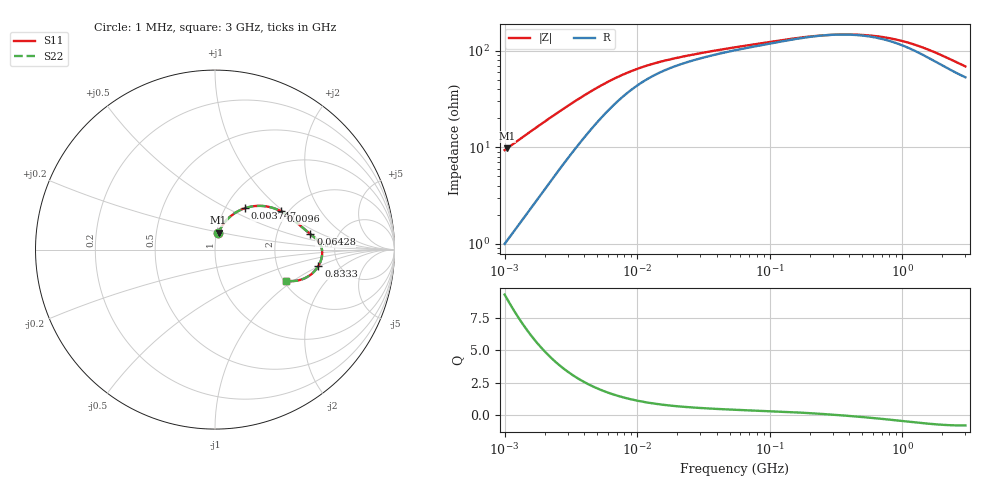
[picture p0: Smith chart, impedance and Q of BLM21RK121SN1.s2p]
! BLM21RK121SN1
# Hz S RI R 50
!Freq.(Hz) S11(Real) S11(Imag) S21(Real) S21(Imag) S12(Real) S12(Imag) S22(Real) S22(Imag)
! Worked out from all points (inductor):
!   401 points, 1 MHz to 3 GHz, reference 50 ohm
!   read as one part in series: L = 1.48 uH near 1.041 MHz
!   highest Q = 9.02 at 1.041 MHz (marker M1), where L = 1.49 uH
!   self-resonance near 308.7 MHz
!   S11 on the Smith chart (normalised r, x): 1 MHz: 1.02, +0.19; 3.747 MHz: 1.23, +0.62; 9.6 MHz: 1.84, +0.96; 64.28 MHz: 3.12, +0.77; 833.3 MHz: 3.50, -0.98; 3 GHz: 2.07, -0.88
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1000000  0.0183 0.0908  0.9817 -0.0908  0.9817 -0.0908  0.0183 0.0908
1040844  0.0197 0.0942  0.9803 -0.0942  0.9803 -0.0942  0.0197 0.0942
1492300  0.0382 0.1296  0.9618 -0.1296  0.9618 -0.1296  0.0382 0.1296
2055611  0.067 0.1668  0.933 -0.1668  0.933 -0.1668  0.067 0.1668
2775447  0.1088 0.2022  0.8912 -0.2022  0.8912 -0.2022  0.1088 0.2022
3747356  0.1662 0.2306  0.8338 -0.2306  0.8338 -0.2306  0.1662 0.2306
3823119  0.1705 0.232  0.8295 -0.232  0.8295 -0.232  0.1705 0.232
4764734  0.2202 0.2425  0.7798 -0.2425  0.7798 -0.2425  0.2202 0.2425
5938264  0.2714 0.2426  0.7286 -0.2426  0.7286 -0.2426  0.2714 0.2426
9600343  0.3682 0.2133  0.6318 -0.2133  0.6318 -0.2133  0.3682 0.2133
1.461624e7  0.4255 0.1754  0.5745 -0.1754  0.5745 -0.1754  0.4255 0.1754
2.509235e7  0.4732 0.1349  0.5268 -0.1349  0.5268 -0.1349  0.4732 0.1349
5.477226e7  0.5225 0.0942  0.4775 -0.0942  0.4775 -0.0942  0.5225 0.0942
6.428402e7  0.5312 0.0872  0.4688 -0.0872  0.4688 -0.0872  0.5312 0.0872
2.094008e8  0.5869 0.0284  0.4131 -0.0284  0.4131 -0.0284  0.5869 0.0284
4.304467e8  0.5968 -0.0277  0.4032 0.0277  0.4032 0.0277  0.5968 -0.0277
8.005644e8  0.5781 -0.088  0.4219 0.088  0.4219 0.088  0.5781 -0.088
8.332625e8  0.5757 -0.0922  0.4243 0.0922  0.4243 0.0922  0.5757 -0.0922
1.218836e9  0.5424 -0.1321  0.4576 0.1321  0.4576 0.1321  0.5424 -0.1321
1.782824e9  0.4893 -0.1641  0.5107 0.1641  0.5107 0.1641  0.4893 -0.1641
2.312676e9  0.4441 -0.1746  0.5559 0.1746  0.5559 0.1746  0.4441 -0.1746
3e9  0.3975 -0.1728  0.6025 0.1728  0.6025 0.1728  0.3975 -0.1728
